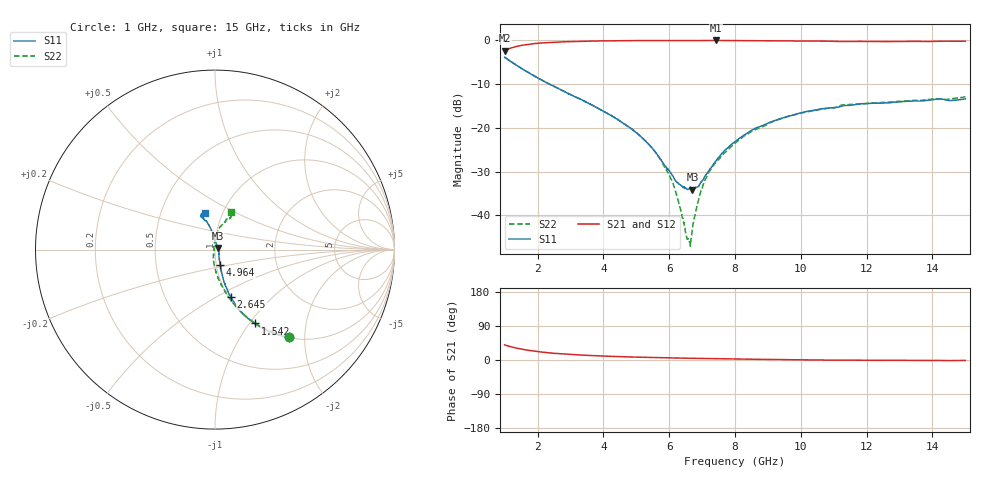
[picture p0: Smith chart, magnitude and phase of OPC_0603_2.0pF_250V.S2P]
! FILE NAME
! DATE 08/20/2012  12:15
! CORRECTED  DATA
# GHz  S  MA  R  50.00
!  FREQ  S11M  S11A  S21M  S21A  S12M  S12A  S22M  S22A
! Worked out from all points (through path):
!   1601 points, 1 GHz to 15 GHz, reference 50 ohm
!   highest |S21| = -0.05 dB at 7.423 GHz (marker M1); lowest = -2.3 dB at 1 GHz (marker M2)
!   group delay of S21, straight-line fit = 5.15 ps
!   lowest |S11| = -34.2 dB at 6.705 GHz (marker M3), VSWR 1.04, Z = 51.8 + j0.884 ohm
!   |S11| at or under -10 dB: 2.351 GHz to end of sweep
!   |S22| runs from -47.1 to -3.9 dB; largest |S21 - S12| = 0.0091
!   S11 on the Smith chart (normalised r, x): 1 GHz: 1.01, -1.67; 1.542 GHz: 1.01, -1.07; 2.645 GHz: 1.02, -0.59; 4.964 GHz: 1.04, -0.18; 15 GHz: 0.82, +0.36
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1  0.6389 -50.0  0.7631 39.8  0.7626 39.8  0.6391 -49.6
1.5425  0.4686 -61.5  0.8773 28.2  0.8762 28.1  0.4688 -61.3
2.645  0.279 -71.4  0.9533 16.7  0.9522 16.7  0.2781 -73.4
3.33625  0.2092 -73.9  0.9723 13.0  0.971 13.0  0.2087 -78.9
4.96375  0.0903 -71.6  0.991 7.6  0.9901 7.6  0.08966 -92.4
5.6725  0.04731 -61.8  0.9925 6.0  0.9918 5.9  0.04685 -101.6
6.13625  0.02683 -37.2  0.9901 5.1  0.9894 5.1  0.02183 -112.2
6.34625  0.02213 -15.1  0.9884 4.8  0.9876 4.8  0.01161 -120.2
6.57375  0.01971 10.0  0.9885 4.6  0.988 4.6  0.005421 -168.5
6.635  0.0205 17.7  0.9881 4.6  0.9873 4.5  0.004803 159.0
6.705  0.01961 25.8  0.9894 4.5  0.9886 4.5  0.007021 143.6
6.8625  0.02103 44.2  0.9907 4.3  0.9897 4.2  0.01353 119.3
7.01125  0.02485 60.7  0.9915 4.1  0.9909 4.0  0.0209 107.8
7.20375  0.03225 74.4  0.9925 3.8  0.9916 3.7  0.03093 99.9
7.4225  0.04178 84.9  0.9941 3.4  0.9921 3.4  0.04043 94.2
8  0.06943 94.7  0.991 2.6  0.9899 2.6  0.06644 89.8
8.56875  0.09627 98.9  0.9887 2.0  0.9876 1.9  0.09298 83.8
9.1375  0.1183 101.5  0.9856 1.4  0.9848 1.3  0.1172 80.0
10.33625  0.157 105.7  0.9794 0.1  0.9782 0.1  0.1556 71.5
11.29875  0.1789 109.6  0.9688 -0.3  0.9677 -0.4  0.1822 68.2
12.6725  0.1921 112.3  0.9638 -0.7  0.9632 -0.8  0.1963 64.3
15  0.2137 105.2  0.9755 -1.2  0.9745 -1.2  0.2264 66.9
